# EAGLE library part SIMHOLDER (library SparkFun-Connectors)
SIM Cellular Card Socket SMT 6 pin standard connection. SparkFun Products: SIM Socket SparkFun Cellular Shield - MG2639 SparkFun SIM Card Socket Breakout
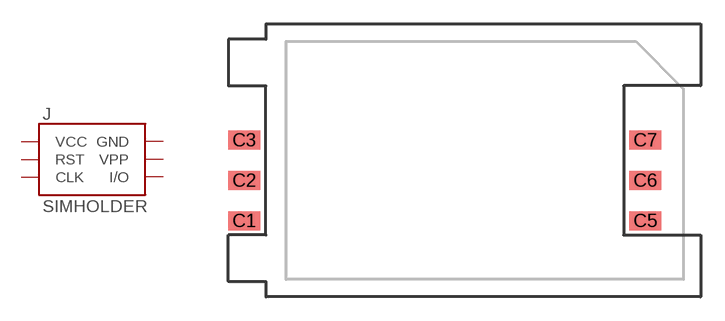
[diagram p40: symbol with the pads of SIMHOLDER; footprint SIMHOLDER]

Designator prefix J

## SIMHOLDERSIM (PROD_ID: CONN-08536; SF_ID: PRT-00548)  [SIMHOLDER]
C1  VCC  pwr
C2  RST  in
C3  CLK  in
C5  GND  pwr
C6  VPP  in
C7  I/O

## Footprint SIMHOLDER (pad centres in mm)
SIM Card Socket SMT Specifications: Pin count: 6 Pin pitch:2.54mm Datasheet referenced for footprint Example device(s): SIMHOLDER
smd 2 x 1.2: C1 -12.61,-3.81; C2 -12.61,-1.27; C3 -12.61,1.27; C5 12.61,-3.81; C6 12.61,-1.27; C7 12.61,1.27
